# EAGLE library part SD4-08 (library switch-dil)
DIL/CODE SWITCH
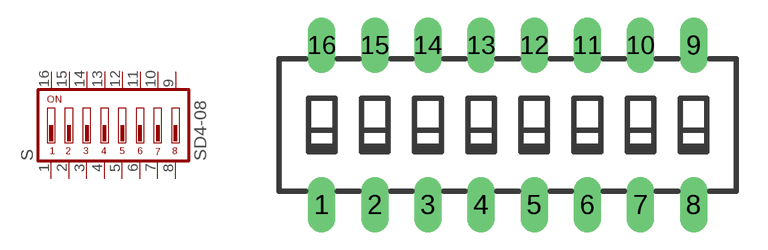
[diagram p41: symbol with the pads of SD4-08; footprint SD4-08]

Designator prefix S

## SD4-08 (OC_FARNELL: unknown; OC_NEWARK: unknown)  [SD4-08]
1  1  pas
2  2  pas
3  3  pas
4  4  pas
5  5  pas
6  6  pas
7  7  pas
8  8  pas
9  9  pas
10  10  pas
11  11  pas
12  12  pas
13  13  pas
14  14  pas
15  15  pas
16  16  pas

## Footprint SD4-08 (pad centres in mm)
DIL/CODE SWITCH Mors
drill 0.813 long: 1 -8.89,-3.81; 2 -6.35,-3.81; 3 -3.81,-3.81; 4 -1.27,-3.81; 5 1.27,-3.81; 6 3.81,-3.81; 7 6.35,-3.81; 8 8.89,-3.81; 9 8.89,3.81; 10 6.35,3.81; 11 3.81,3.81; 12 1.27,3.81; 13 -1.27,3.81; 14 -3.81,3.81; 15 -6.35,3.81; 16 -8.89,3.81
